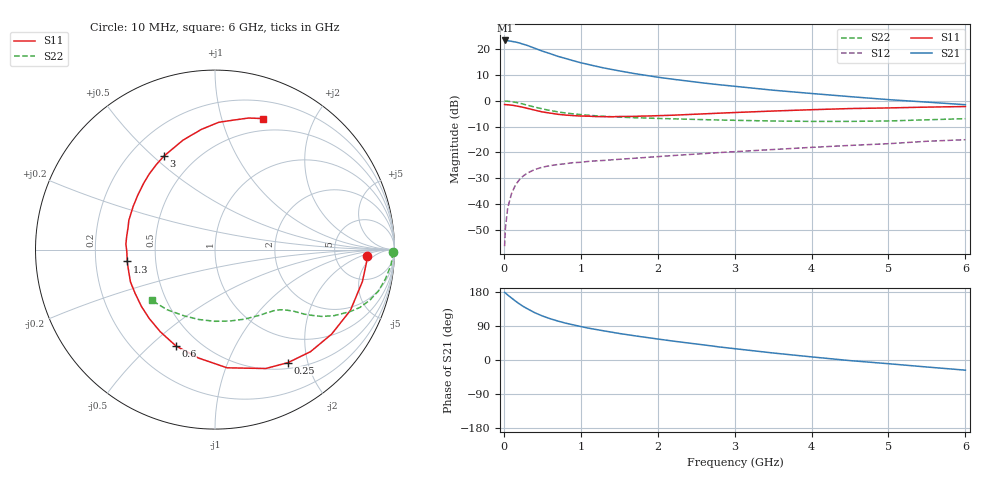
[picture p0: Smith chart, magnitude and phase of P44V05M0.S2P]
! SIEMENS Small Signal Semiconductors
! BFP182
! Si NPN RF Bipolar Junction Transistor in SOT143
! VCE = 4 V  IC = 5 mA
! Common Emitter S-Parameters:  March  1996
# GHz  S  MA  R  50
!  f  S11  S21  S12  S22
! GHz  MAG  ANG  MAG  ANG  MAG  ANG  MAG  ANG
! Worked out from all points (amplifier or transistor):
!   36 points, 10 MHz to 6 GHz, reference 50 ohm
!   highest |S21| = 23.5 dB at 20 MHz (marker M1)
!   |S21| within 3 dB of that: start of sweep to 399.1 MHz
!   unconditionally stable (mu >= 1): 1.614 GHz to 5.579 GHz
!   at 250 MHz: K = 0.21, MSG = 25.6 dB, |S12| = -29.2 dB
!   at 1.4 GHz: K = 0.92, MSG = 17.6 dB, |S12| = -22.9 dB
!   at 6 GHz: K = 0.96, MSG = 6.8 dB, |S12| = -15.1 dB
!   lowest NFmin = 1.20 dB at 450 MHz
!   S11 on the Smith chart (normalised r, x): 10 MHz: 11, -3; 250 MHz: 0.59, -1.68; 600 MHz: 0.38, -0.61; 1.3 GHz: 0.34, -0.06; 3 GHz: 0.34, +0.54; 6 GHz: 0.37, +1.36
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0.01  0.8481 -2.4  14.81 178.4  0.0015 84.4  0.9914 -0.9
0.02  0.8469 -5.0  14.95 177.0  0.0033 89.4  0.9896 -2.0
0.05  0.8404 -12.2  14.81 171.6  0.0083 84.5  0.9846 -5.0
0.1  0.827 -24.1  14.37 163.6  0.0158 76.4  0.9638 -9.7
0.15  0.8025 -35.9  13.96 155.7  0.023 71.6  0.9389 -14.3
0.2  0.7788 -46.9  13.39 148.4  0.0292 66.1  0.9065 -18.2
0.25  0.7497 -57.1  12.67 141.6  0.0345 61.3  0.8688 -21.8
0.3  0.7203 -66.9  12.04 135.9  0.0391 57.2  0.8289 -24.6
0.4  0.662 -84.2  10.57 125.0  0.0463 50.4  0.7591 -29.0
0.5  0.6104 -98.9  9.285 116.3  0.0514 45.6  0.7005 -32.1
0.6  0.5792 -112.1  8.309 109.1  0.0551 42.0  0.6514 -34.2
0.7  0.5497 -123.8  7.361 102.9  0.0579 39.5  0.6127 -35.9
0.8  0.5306 -133.7  6.691 97.4  0.0601 37.4  0.5828 -37.0
1.1  0.5043 -159.0  5.101 84.0  0.0667 34.5  0.5255 -40.0
1.3  0.4936 -172.3  4.37 76.9  0.0696 33.6  0.5018 -41.9
1.7  0.4999 165.6  3.391 63.9  0.0768 33.2  0.4709 -46.4
2.2  0.5268 144.6  2.634 49.9  0.0866 32.9  0.4483 -53.4
3  0.594 118.5  1.923 29.9  0.103 31.1  0.4193 -67.8
3.5  0.6353 106.3  1.614 18.5  0.1134 29.1  0.4063 -78.4
4.5  0.7097 88.3  1.21 -1.6  0.1363 24.4  0.3996 -102.9
5.5  0.7568 75.6  0.947 -18.5  0.1642 19.3  0.4288 -128.7
6  0.777 70.0  0.843 -26.8  0.1761 15.0  0.4515 -141.2
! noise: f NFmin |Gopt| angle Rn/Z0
0.45  1.2  0.27  37  0.3
0.9  1.3  0.25  75  0.23
1.8  1.9  0.21  145  0.2
